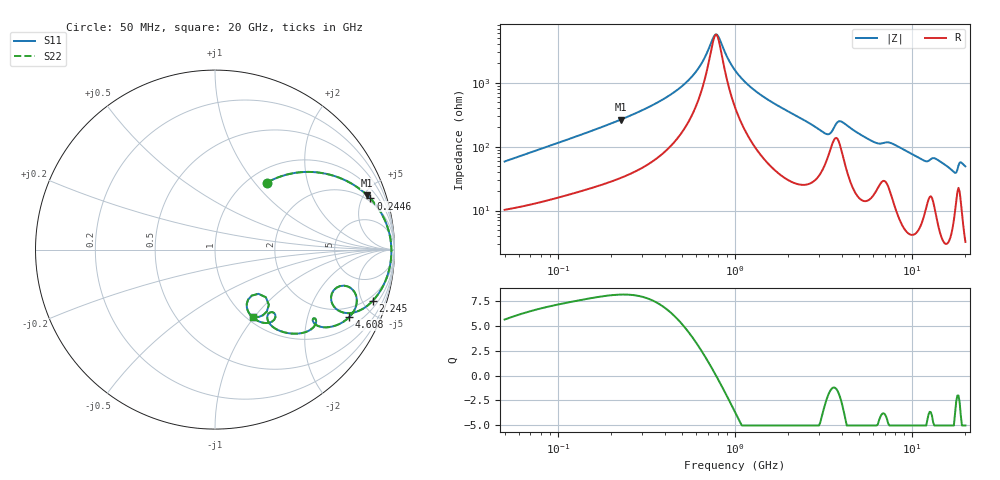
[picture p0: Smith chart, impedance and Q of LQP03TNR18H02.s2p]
!Murata Part Number: LQP03TNR18H02
!These Parameters are Measured in Series Mode Connection
!  o--[Z]--o
!Port1  Port2
!  o-------o
!Freq. Start=50[MHz] Stop=20[GHz], 401[Steps]
# Hz S RI R 50
!Freq.(Hz) S11(Real) S11(Imag) S21(Real) S21(Imag) S12(Real) S12(Imag) S22(Real) S22(Imag)
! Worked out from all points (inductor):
!   401 points, 50 MHz to 20 GHz, reference 50 ohm
!   read as one part in series: L = 181 nH near 51.52 MHz
!   highest Q = 8.11 at 227 MHz (marker M1), where L = 185 nH
!   self-resonance near 775.2 MHz
!   S11 on the Smith chart (normalised r, x): 50 MHz: 1.21, +1.15; 244.6 MHz: 1.71, +5.75; 2.245 GHz: 1.52, -5.94; 4.608 GHz: 1.46, -3.68; 20 GHz: 1.06, -0.98
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5e7  0.2881 0.3725  0.7119 -0.3725  0.7119 -0.3725  0.2881 0.3725
1.364002e8  0.6845 0.4034  0.3155 -0.4034  0.3155 -0.4034  0.6845 0.4034
2.269813e8  0.8477 0.3029  0.1523 -0.3029  0.1523 -0.3029  0.8477 0.3029
2.446335e8  0.8657 0.2848  0.1343 -0.2848  0.1343 -0.2848  0.8657 0.2848
3.721004e8  0.9391 0.1794  0.0609 -0.1794  0.0609 -0.1794  0.9391 0.1794
5.745257e8  0.9751 0.0729  0.0249 -0.0729  0.0249 -0.0729  0.9751 0.0729
7.751977e8  0.9827 0.00182  0.0173 -0.00182  0.0173 -0.00182  0.9827 0.00182
8.108264e8  0.9828 -0.00885  0.0172 0.00885  0.0172 0.00885  0.9828 -0.00885
1e9  0.9798 -0.0594  0.0202 0.0594  0.0202 0.0594  0.9798 -0.0594
1.349283e9  0.9636 -0.1359  0.0364 0.1359  0.0364 0.1359  0.9636 -0.1359
2.245319e9  0.8787 -0.2855  0.1213 0.2855  0.1213 0.2855  0.8787 -0.2855
2.728004e9  0.7986 -0.3424  0.2014 0.3424  0.2014 0.3424  0.7986 -0.3424
3.265178e9  0.6624 -0.3171  0.3376 0.3171  0.3376 0.3171  0.6624 -0.3171
3.680849e9  0.7181 -0.2008  0.2819 0.2008  0.2819 0.2008  0.7181 -0.2008
4.608136e9  0.7488 -0.3753  0.2512 0.3753  0.2512 0.3753  0.7488 -0.3753
6.311513e9  0.554 -0.412  0.446 0.412  0.446 0.412  0.554 -0.412
7.442007e9  0.5614 -0.4116  0.4386 0.4116  0.4386 0.4116  0.5614 -0.4116
1.131968e10  0.3043 -0.4127  0.6957 0.4127  0.6957 0.4127  0.3043 -0.4127
1.460232e10  0.2603 -0.4056  0.7397 0.4056  0.7397 0.4056  0.2603 -0.4056
1.747767e10  0.1842 -0.279  0.8158 0.279  0.8158 0.279  0.1842 -0.279
1.855685e10  0.3002 -0.3075  0.6998 0.3075  0.6998 0.3075  0.3002 -0.3075
2e10  0.2093 -0.3752  0.7907 0.3752  0.7907 0.3752  0.2093 -0.3752
